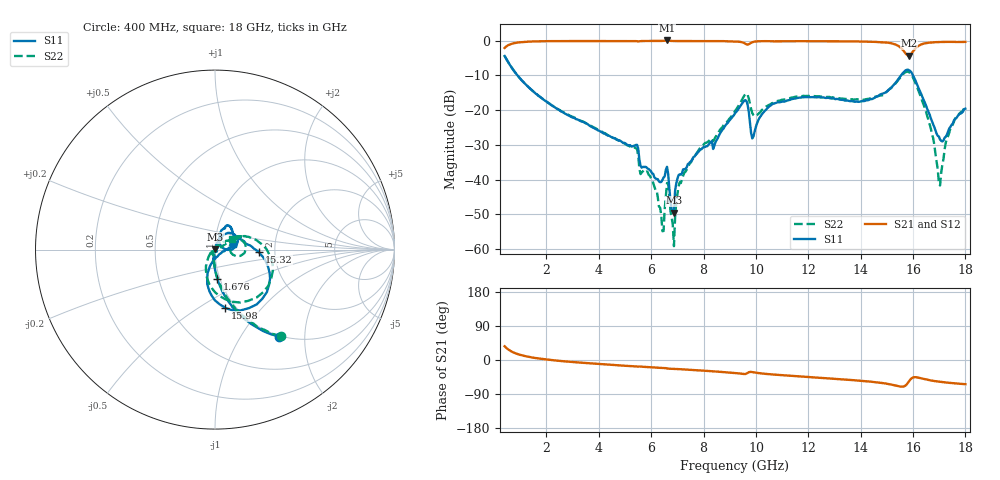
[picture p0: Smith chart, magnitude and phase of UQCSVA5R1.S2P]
!  Part Number  UQCSVA5R1  Mounting Orientation: Horizontal
!  Description: Ultra Low ESR Microwave capacitors
!  Application: Coupling, Bypass, Tuning, DC Block
!  Filters, Matching
# GHZ S DB R 50
! Freq  |S11|  S11 Ph  |S21|  S21 Ph  |S12|  S12 Ph  |S22|  S22 Ph
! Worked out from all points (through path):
!   401 points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, 400 MHz to 18 GHz, reference 50 ohm
!   highest |S21| = 0.09 dB at 6.604 GHz (marker M1); lowest = -4.3 dB at 15.84 GHz (marker M2)
!   group delay of S21, straight-line fit = 12.2 ps
!   lowest |S11| = -49.6 dB at 6.868 GHz (marker M3), VSWR 1.01, Z = 50.3 + j0.183 ohm
!   |S11| at or under -10 dB: 892.8 MHz to 15.54 GHz (14.65 GHz wide, 178 % of centre); 16 GHz to end of sweep
!   |S22| runs from -59.2 to -4.4 dB; largest |S21 - S12| = 0.0085
!   S11 on the Smith chart (normalised r, x): 400 MHz: 0.98, -1.50; 1.676 GHz: 0.97, -0.32; 15.32 GHz: 1.65, -0.05; 15.98 GHz: 0.90, -0.66; 18 GHz: 1.22, +0.07
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0.4  -4.40 -53.6  -2.08 36.2  -2.08 36.2  -4.36 -52.8
1.676  -15.79 -85.5  -0.17 4.2  -0.18 4.1  -15.70 -84.3
3.348  -23.28 -95.8  -0.08 -7.2  -0.08 -7.2  -23.17 -94.3
5.372  -30.22 -99.7  -0.08 -17.1  -0.08 -17.0  -30.76 -118.4
6.296  -40.56 -55.6  -0.05 -20.6  -0.05 -20.4  -47.84 -124.6
6.428  -40.14 -41.1  -0.04 -21.0  -0.03 -20.9  -54.92 -149.7
6.604  -36.34 -54.4  0.09 -22.2  0.09 -22.0  -41.02 12.4
6.868  -49.60 33.4  -0.08 -23.6  -0.08 -23.5  -59.22 49.5
7.352  -36.57 36.1  -0.07 -25.4  -0.07 -25.2  -37.19 62.8
9.2  -20.91 61.3  -0.20 -34.2  -0.19 -34.0  -20.26 31.5
9.596  -17.11 30.2  -0.85 -36.8  -0.84 -36.6  -15.36 11.1
9.904  -27.56 49.5  -0.32 -32.3  -0.30 -32.1  -21.43 -4.0
10.608  -18.38 69.5  -0.15 -38.1  -0.14 -38.0  -18.01 25.7
12.148  -16.24 58.5  -0.14 -45.5  -0.14 -45.3  -15.97 26.7
15.096  -13.93 5.8  -0.62 -63.9  -0.61 -63.6  -13.99 20.9
15.316  -12.22 -3.1  -1.05 -67.1  -1.03 -66.7  -12.45 12.4
15.844  -8.48 -60.1  -4.26 -56.4  -4.24 -56.1  -9.03 -49.1
15.976  -9.62 -79.8  -3.29 -46.9  -3.27 -46.7  -10.28 -71.6
16.592  -20.51 -106.8  -0.57 -52.9  -0.56 -52.6  -22.88 -125.9
16.988  -27.61 -73.2  -0.37 -57.2  -0.36 -56.8  -41.05 174.7
17.384  -25.25 -8.1  -0.32 -60.3  -0.31 -60.0  -26.47 46.3
18  -19.58 16.5  -0.32 -63.8  -0.31 -63.5  -19.24 32.4
